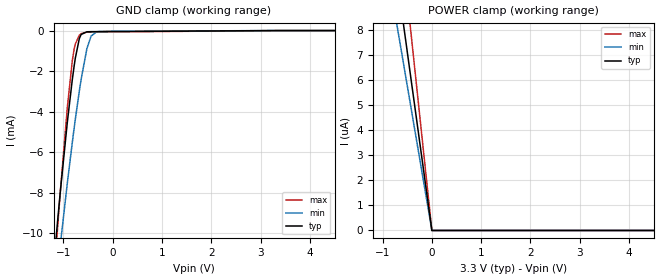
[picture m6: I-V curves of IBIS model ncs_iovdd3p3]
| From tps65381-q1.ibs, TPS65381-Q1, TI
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|   ncs_iovdd3p3 Model
[Model]   ncs_iovdd3p3
Model_type   Input
Vinl = 0.99
Vinh = 2.31
|   typ   min   max
|   (nom PVT)   (fast PVT)   (slow PVT)
C_comp   5.965e-13   4.988e-13   6.512e-13
[Model spec]
|subparameter
Vinl   0.99   0.951   1.029
Vinh   2.31   2.219   2.401
| Where nom  PVT is Nominal Process, 3.3V, 27C
|   Fast PVT is Strong Process,  3.43V, -40C
|   Slow PVT is Weak Process,   3.17V, 150C
[Voltage Range]   3.3   3.17   3.43
|Junction Temperature
[Temperature Range]   27   150   -40
[Power Clamp Reference]   3.3   3.17   3.43
[GND Clamp Reference]   0   0   0
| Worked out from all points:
|   GND clamp passes 1 mA (typ) near -0.73 V on its own axis
[GND Clamp]
|   Voltage   I(typ)   I(min)   I(max)
-3.3V     -92.24mA   -77.03mA   -111.9mA
-1.228V   -12.43mA   -14.36mA   -13.43mA
-1.119V   -9.44mA    -11.84mA   -9.768mA
-1.059V   -7.877mA   -10.5mA    -7.86mA
-923mV    -4.589mA   -7.587mA   -3.885mA
-820.1mV  -2.44mA    -5.535mA   -1.505mA
-758.4mV  -1.363mA   -4.384mA   -661.7uA
-640.2mV  -193.6uA   -2.407mA   -147.2uA
-523.1mV  -59.15uA   -886.9uA   -76.34uA
-437.5mV  -53.68uA   -271.1uA   -72.02uA
-301.2mV  -51.41uA   -53.03uA   -69.35uA
6.6V      0A         0A         0A
[POWER Clamp]
|   Voltage   I(typ)   I(min)   I(max)
-3.3V     47.11uA    38.15uA    61.34uA
-1.119V   15.97uA    12.94uA    20.8uA
-330mV    4.711uA    3.819uA    6.134uA
-340uV    0A         0A         0A
6.6V      0A         0A         0A
